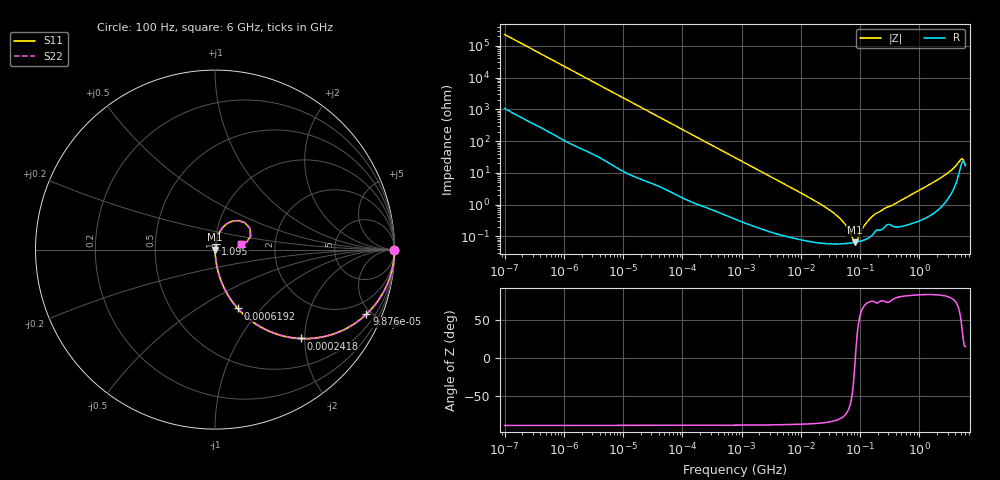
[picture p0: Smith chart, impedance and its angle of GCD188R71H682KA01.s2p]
!Murata Part Number: GCD188R71H682KA01
!These Parameters are Measured in Series Mode Connection
!Data Generated on Mar 13, 2026
!  o--ll--o
!Port1  Port2
!  o------o
!Operation Temp=25[degC], DC Bias Voltage=0[V]
!Freq. Start=100[Hz] Stop=6[GHz] 401[Steps]
# Hz S RI R 50
!Freq.(Hz) S11(Real) S11(Imag) S21(Real) S21(Imag) S12(Real) S12(Imag) S22(Real) S22(Imag)
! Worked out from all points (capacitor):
!   401 points, 100 Hz to 6 GHz, reference 50 ohm
!   read as one part in series: C = 7.03 nF near 109 Hz
!   lowest |Z| = 66.2 mohm at 81.54 MHz (marker M1)
!   series resonance near 83.27 MHz, so ESL is about 520 pH
!   S11 on the Smith chart (normalised r, x): 100 Hz: open; 98.76 kHz: 1.03, -4.68; 241.8 kHz: 1.02, -1.92; 619.2 kHz: 1.01, -0.75; 1.095 GHz: 1.01, +0.06; 6 GHz: 1.34, +0.09
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100  1 -0.000442  2.3e-06 0.000442  2.3e-06 0.000442  1 -0.000442
2008  0.9999 -0.0088  0.000121 0.0088  0.000121 0.0088  0.9999 -0.0088
12592  0.9967 -0.0547  0.00327 0.0547  0.00327 0.0547  0.9967 -0.0547
40335  0.9692 -0.1695  0.0308 0.1695  0.0308 0.1695  0.9692 -0.1695
98762  0.844 -0.3593  0.156 0.3593  0.156 0.3593  0.844 -0.3593
241822  0.4797 -0.4953  0.5203 0.4953  0.5203 0.4953  0.4797 -0.4953
619225  0.1271 -0.3277  0.8729 0.3277  0.8729 0.3277  0.1271 -0.3277
774597  0.0861 -0.2748  0.9139 0.2748  0.9139 0.2748  0.0861 -0.2748
2594782  0.00965 -0.0897  0.9903 0.0897  0.9903 0.0897  0.00965 -0.0897
1.555665e7  0.00089 -0.0148  0.9991 0.0148  0.9991 0.0148  0.00089 -0.0148
4.556224e7  0.000599 -0.00369  0.9994 0.00369  0.9994 0.00369  0.000599 -0.00369
5.960426e7  0.000607 -0.00196  0.9994 0.00196  0.9994 0.00196  0.000607 -0.00196
8.154455e7  0.000651 -0.000119  0.9993 0.000119  0.9993 0.000119  0.000651 -0.000119
8.918374e7  0.000673 0.000398  0.9993 -0.000398  0.9993 -0.000398  0.000673 0.000398
1.166697e8  0.000777 0.00199  0.9992 -0.00199  0.9992 -0.00199  0.000777 0.00199
1.526266e8  0.00102 0.00376  0.999 -0.00376  0.999 -0.00376  0.00102 0.00376
3.124326e8  0.00244 0.00839  0.9976 -0.00839  0.9976 -0.00839  0.00244 0.00839
1.094528e9  0.00423 0.0308  0.9958 -0.0308  0.9958 -0.0308  0.00423 0.0308
3.352442e9  0.0316 0.1077  0.9684 -0.1077  0.9684 -0.1077  0.0316 0.1077
4.796499e9  0.134 0.1613  0.866 -0.1613  0.866 -0.1613  0.134 0.1613
5.245841e9  0.194 0.119  0.806 -0.119  0.806 -0.119  0.194 0.119
6e9  0.1454 0.0329  0.8546 -0.0329  0.8546 -0.0329  0.1454 0.0329
